(* Logix 5000 AddOnInstructionDefinition export NXEE2_Generic_Apply_Preset; software revision 20.03 *)

ADD_ON_INSTRUCTION NXEE2_Generic_Apply_Preset   (* revision 1.0, vendor AMCI, ExecuteEnableInFalse *)
// Revision note:
// 1/29/21 V1.0 is the initial release
VAR_INPUT
   Ch1_Status_Word : INT; {required}
        .0   // set when command error
        .2   // set when reference voltage error
        .3   // set when reference frequency error
        .4   // command error
        .5   // config error
        .6   // setup error
        .7   // scalar errors
        .8   // preset value error
        .9   // full scale count error
        .15   // ACK bit
   ch2_Status_Word : INT; {required}
        .4   // command error
        .5   // config error
        .6   // setup error
        .7   // scalar errors
        .8   // preset value error
        .9   // full scale count error
   Apply_Preset_Ch1_0_NO_1_YES : BOOL; {required}
   Apply_Preset_Ch2_0_NO_1_YES : BOOL; {required}
   save_in_flash_0_NO_1_YES : BOOL; {required}
END_VAR
VAR_OUTPUT
   EN : BOOL; {access Read Only, visible}
   DN : BOOL; {access Read Only, visible}
   ER : BOOL; {visible}
END_VAR
VAR_IN_OUT
   AMCI_NXEE2_output_data : INT[10]; {required}
END_VAR
VAR
   command_data_block : INT[10];
        [0]   // Command Word
        [0].15   // Transmit bit
        [1]   // Setup Word
        [2]   // channel 1 Full Scale_Count
        [3]   // channel 1 Preset Value
        [4]   // channel 1 Transformation Ratio
        [5]   // channel 2 Full Scale Count
        [6]   // channel 2 Preset Value
        [7]   // channel 2 Transformation Ratio
        [8]   // Reference Voltage
        [9]   // Reference Frequency
   Allow_Programming : BOOL; {access None}
END_VAR

ROUTINE EnableInFalse   (* ladder *)
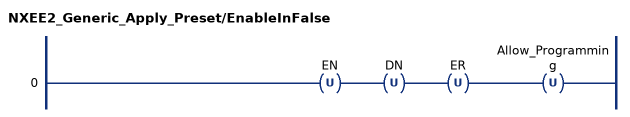
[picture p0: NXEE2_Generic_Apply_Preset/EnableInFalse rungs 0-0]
   0: OTU(EN)OTU(DN)OTU(ER)OTU(Allow_Programming);
END_ROUTINE

ROUTINE Logic   (* ladder *)
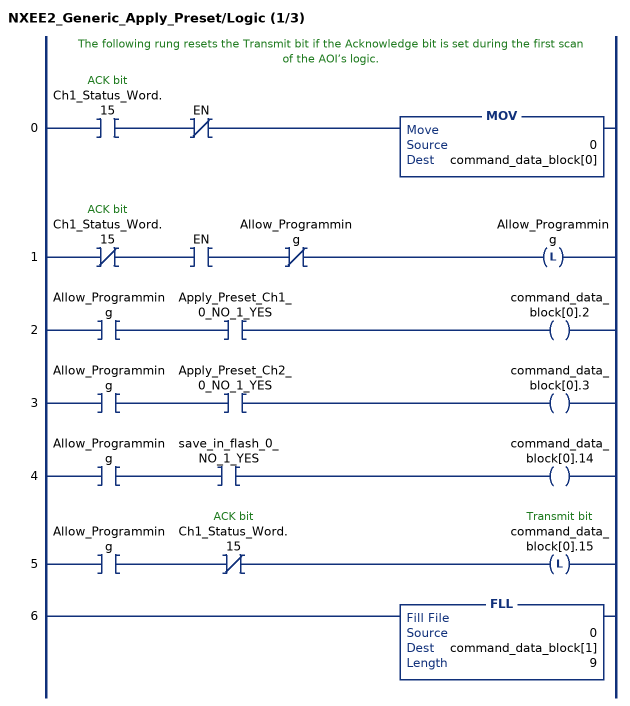
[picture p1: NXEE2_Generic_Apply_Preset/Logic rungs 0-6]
   // The following rung resets the Transmit bit if the Acknowledge bit is set during the first scan of the AOI’s logic.
   0: XIC(Ch1_Status_Word.15)XIO(EN)MOV(0,command_data_block[0]);
   1: XIO(Ch1_Status_Word.15)XIC(EN)XIO(Allow_Programming)OTL(Allow_Programming);
   2: XIC(Allow_Programming)XIC(Apply_Preset_Ch1_0_NO_1_YES)OTE(command_data_block[0].2);
   3: XIC(Allow_Programming)XIC(Apply_Preset_Ch2_0_NO_1_YES)OTE(command_data_block[0].3);
   4: XIC(Allow_Programming)XIC(save_in_flash_0_NO_1_YES)OTE(command_data_block[0].14);
   5: XIC(Allow_Programming)XIO(Ch1_Status_Word.15)OTL(command_data_block[0].15);
   6: FLL(0,command_data_block[1],9);
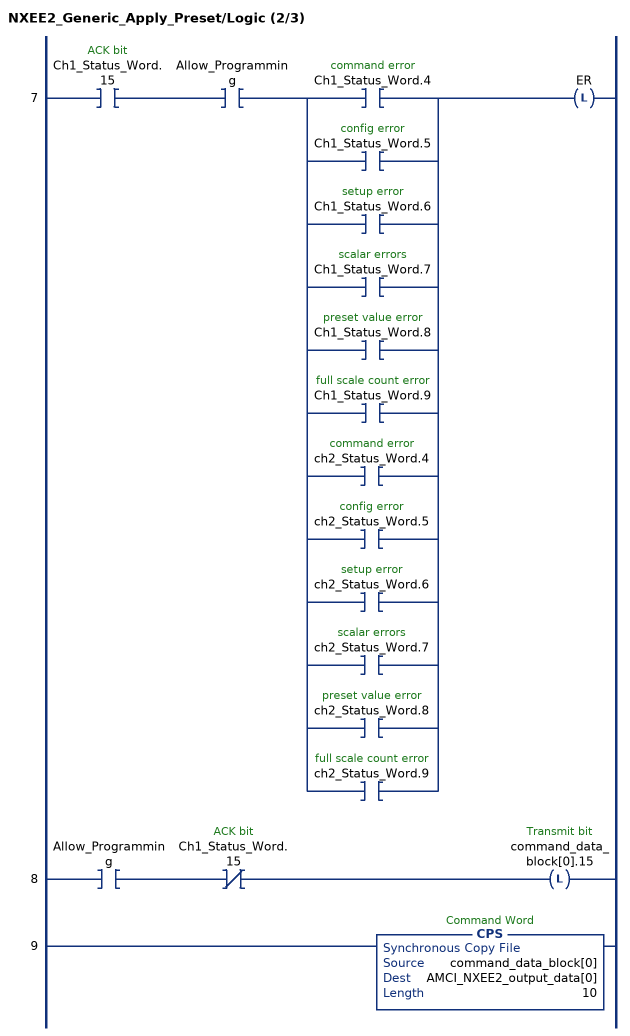
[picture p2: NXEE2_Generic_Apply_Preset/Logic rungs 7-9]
   7: XIC(Ch1_Status_Word.15)XIC(Allow_Programming)[XIC(Ch1_Status_Word.4) ,XIC(Ch1_Status_Word.5) ,XIC(Ch1_Status_Word.6) ,XIC(Ch1_Status_Word.7) ,XIC(Ch1_Status_Word.8) ,XIC(Ch1_Status_Word.9) ,XIC(ch2_Status_Word.4) ,XIC(ch2_Status_Word.5) ,XIC(ch2_Status_Word.6) ,XIC(ch2_Status_Word.7) ,XIC(ch2_Status_Word.8) ,XIC(ch2_Status_Word.9) ]OTL(ER);
   8: XIC(Allow_Programming)XIO(Ch1_Status_Word.15)OTL(command_data_block[0].15);
   9: CPS(command_data_block[0],AMCI_NXEE2_output_data[0],10);
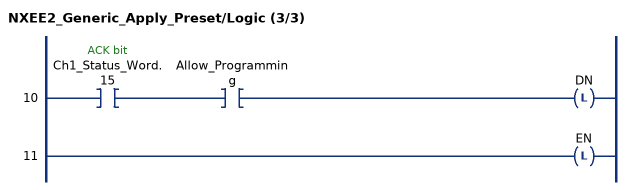
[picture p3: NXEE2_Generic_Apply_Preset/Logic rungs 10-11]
   10: XIC(Ch1_Status_Word.15)XIC(Allow_Programming)OTL(DN);
   11: OTL(EN);
END_ROUTINE
END_ADD_ON_INSTRUCTION
